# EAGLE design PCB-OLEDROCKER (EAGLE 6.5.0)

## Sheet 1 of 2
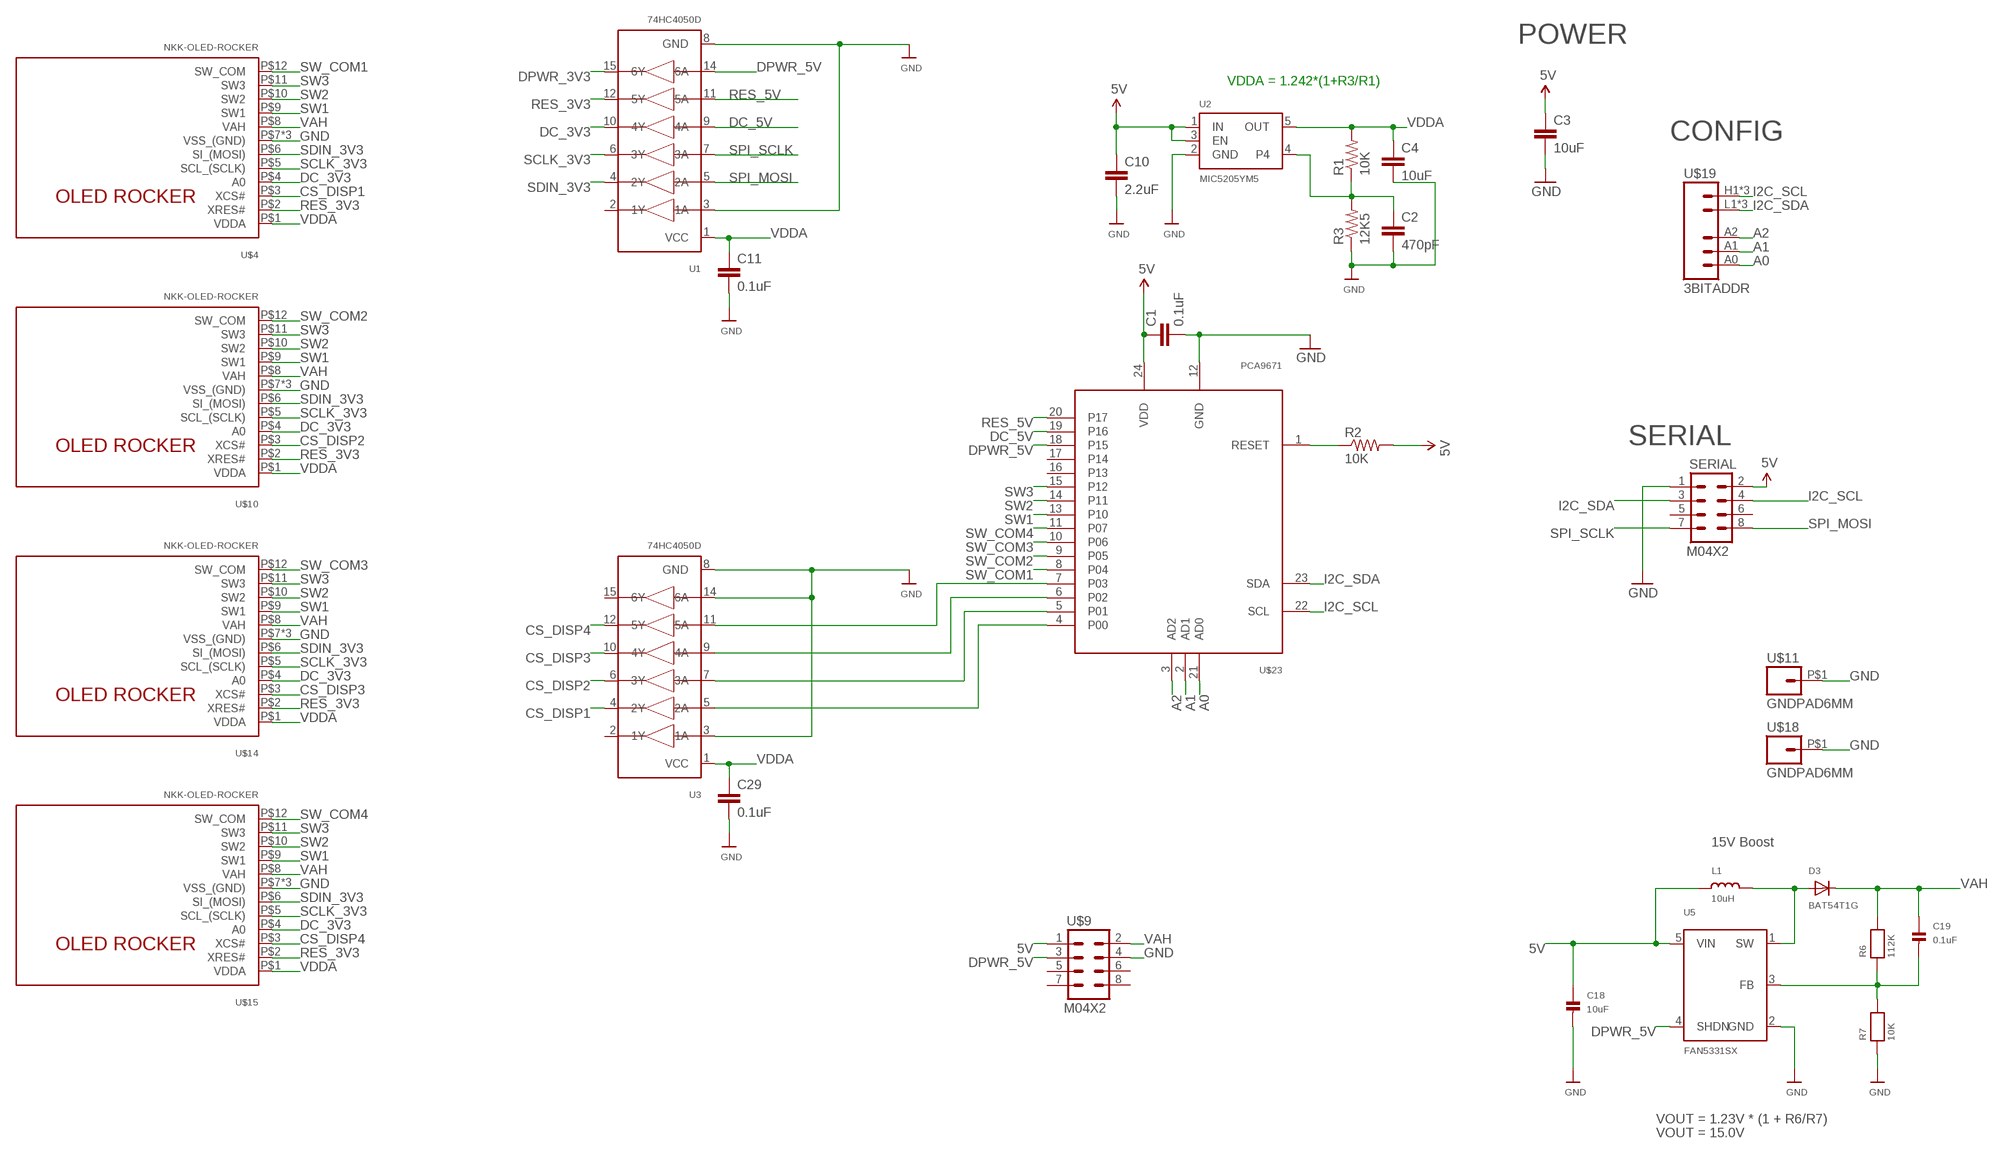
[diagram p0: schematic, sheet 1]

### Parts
C1  0.1uF  CAP0603-CAP  [0603-CAP]
C2  470pF  CAP0603-CAP  [0603-CAP]
C3  10uF  CAP0805  [0805]
C4  10uF  CAP0805  [0805]
C10  2.2uF  CAP0603-CAP  [0603-CAP]
C11  0.1uF  CAP0603-CAP  [0603-CAP]
C18  10uF  CAP_CERAMIC0805  [0805]
C19  0.1uF  CAP_CERAMIC0603  [0603]
C29  0.1uF  CAP0603-CAP  [0603-CAP]
D3  BAT54T1G  DIODESOD-123  [SOD-123]
L1  10uH  INDUCTOR  [INDUCTOR_1007]
R1  10K  RESISTOR0603-RES  [0603-RES]
R2  10K  RESISTOR0603-RES  [0603-RES]
R3  12K5  RESISTOR0603-RES  [0603-RES]
R6  112K  RESISTOR0603  [0603]
R7  10K  RESISTOR0603  [0603]
SERIAL  M04X2  [2X4]
U1  74HC4050D  74HC4050DTSSOP16  [TSSOP16]
U2  MIC5205YM5  VREG_SOT23-5  [SOT23-5]
U3  74HC4050D  74HC4050DTSSOP16  [TSSOP16]
U5  FAN5331SX  FAN5331  [SOT23-5]
U$4  NKK-OLED-ROCKER  [JST_BM12B-SURS]
U$9  M04X2  [2X4]
U$10  NKK-OLED-ROCKER  [JST_BM12B-SURS]
U$11  GNDPAD6MM  [3.2MMPAD6MM]
U$14  NKK-OLED-ROCKER  [JST_BM12B-SURS]
U$15  NKK-OLED-ROCKER  [JST_BM12B-SURS]
U$18  GNDPAD6MM  [3.2MMPAD6MM]
U$19  3BITADDR  [3BITADDR]
U$23  PCA9671  [TSSOP24]

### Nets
5V [Power]: C1.1 C3.1 C10.1 C18.1 L1.P$1 R2.2 SERIAL.2 U2.1(IN) U2.3(EN) U5.5(VIN) U$9.1 U$23.24(VDD)
A0: U$19.A0 U$23.21(AD0)
A1: U$19.A1 U$23.2(AD1)
A2: U$19.A2 U$23.3(AD2)
CS_DISP1: U3.4(2Y) U$4.P$3(XCS#)
CS_DISP2: U3.6(3Y) U$10.P$3(XCS#)
CS_DISP3: U3.10(4Y) U$14.P$3(XCS#)
CS_DISP4: U3.12(5Y) U$15.P$3(XCS#)
DC_3V3: U1.10(4Y) U$4.P$4(A0) U$10.P$4(A0) U$14.P$4(A0) U$15.P$4(A0)
DC_5V: U1.9(4A) U$23.19(P16)
DPWR_3V3: U1.15(6Y)
DPWR_5V [Power]: U1.14(6A) U5.4(SHDN) U$9.3 U$23.18(P15)
GND [Power]: C1.2 C2.2 C3.2 C4.2 C10.2 C11.2 C18.2 C29.2 R3.1 R7.1 SERIAL.1 U1.3(1A) U1.8(GND) U2.2(GND) U3.3(1A) U3.8(GND) U3.14(6A) U5.2(GND) U$4.P$7(VSS_(GND)) U$4.SUPPORT1(VSS_(GND)) U$4.SUPPORT2(VSS_(GND)) U$9.4 U$10.P$7(VSS_(GND)) U$10.SUPPORT1(VSS_(GND)) U$10.SUPPORT2(VSS_(GND)) U$11.P$1 U$14.P$7(VSS_(GND)) U$14.SUPPORT1(VSS_(GND)) U$14.SUPPORT2(VSS_(GND)) U$15.P$7(VSS_(GND)) U$15.SUPPORT1(VSS_(GND)) U$15.SUPPORT2(VSS_(GND)) U$18.P$1 U$23.12(GND)
I2C_SCL: SERIAL.4 U$19.H1(VCC) U$19.H2(VCC) U$19.H3(VCC) U$23.22(SCL)
I2C_SDA: SERIAL.3 U$19.L1(GND) U$19.L2(GND) U$19.L3(GND) U$23.23(SDA)
N$1: R2.1 U$23.1(RESET)
N$3: C2.1 R1.1 R3.2 U2.4
N$14 [Power]: D3.A L1.P$2 U5.1(SW)
N$15: C19.2 R6.1 R7.2 U5.3(FB)
N$29: U3.5(2A) U$23.4(P00)
N$30: U3.7(3A) U$23.5(P01)
N$31: U3.9(4A) U$23.6(P02)
N$32: U3.11(5A) U$23.7(P03)
RES_3V3: U1.12(5Y) U$4.P$2(XRES#) U$10.P$2(XRES#) U$14.P$2(XRES#) U$15.P$2(XRES#)
RES_5V: U1.11(5A) U$23.20(P17)
SCLK_3V3: U1.6(3Y) U$4.P$5(SCL_(SCLK)) U$10.P$5(SCL_(SCLK)) U$14.P$5(SCL_(SCLK)) U$15.P$5(SCL_(SCLK))
SDIN_3V3: U1.4(2Y) U$4.P$6(SI_(MOSI)) U$10.P$6(SI_(MOSI)) U$14.P$6(SI_(MOSI)) U$15.P$6(SI_(MOSI))
SPI_MOSI: SERIAL.8 U1.5(2A)
SPI_SCLK: SERIAL.7 U1.7(3A)
SW1: U$4.P$9(SW1) U$10.P$9(SW1) U$14.P$9(SW1) U$15.P$9(SW1) U$23.13(P10)
SW2: U$4.P$10(SW2) U$10.P$10(SW2) U$14.P$10(SW2) U$15.P$10(SW2) U$23.14(P11)
SW3: U$4.P$11(SW3) U$10.P$11(SW3) U$14.P$11(SW3) U$15.P$11(SW3) U$23.15(P12)
SW_COM1 [Power]: U$4.P$12(SW_COM) U$23.8(P04)
SW_COM2: U$10.P$12(SW_COM) U$23.9(P05)
SW_COM3: U$14.P$12(SW_COM) U$23.10(P06)
SW_COM4: U$15.P$12(SW_COM) U$23.11(P07)
VAH [Power]: C19.1 D3.C R6.2 U$4.P$8(VAH) U$9.2 U$10.P$8(VAH) U$14.P$8(VAH) U$15.P$8(VAH)
VDDA: C4.1 C11.1 C29.1 R1.2 U1.1(VCC) U2.5(OUT) U3.1(VCC) U$4.P$1(VDDA) U$10.P$1(VDDA) U$14.P$1(VDDA) U$15.P$1(VDDA)
Unconnected: SERIAL.5 SERIAL.6 U1.2(1Y) U3.2(1Y) U3.15(6Y) U$9.5 U$9.6 U$9.7 U$9.8 U$23.16(P13) U$23.17(P14)

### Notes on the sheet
- POWER
- VDDA = 1.242*(1+R3/R1)
- CONFIG
- SERIAL
- 15V Boost
- VOUT = 1.23V * (1 + R6/R7)
- VOUT = 15.0V

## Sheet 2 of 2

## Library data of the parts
C1-C4 C10 C11 C29 = SparkFun:CAP: Capacitor
C18 C19 = microbuilder:CAP_CERAMIC: Ceramic Capacitors
D3 = microbuilder:DIODE: Diode
L1 = microbuilder:INDUCTOR: Inductors
R1-R3 = SparkFun:RESISTOR: Resistor
R6 R7 = microbuilder:RESISTOR: Resistors
SERIAL U$9 = SparkFun:M04X2
U1 U3 = SKAARHOJ:74HC4050D: 6-channel level shifter 74HC4050D - 2V-6V Supply Digikey: 74HC4050D,653-ND Mouser: 771-74HC4050D-T
U2 = microbuilder:VREG_SOT23-5: SOT23-5 Fixed Voltage Regulators To better organise some of the SOT23-5 fixed voltage regulators in this library, this new part was created. Part Current Out V Out V In V Dropout Digikey Part No. ADP121 150mA 3.3V 3.4-5.5V 0.09V @ 150mA ADP121-AUJZ33R7CT-ND ADP121 150mA 3.0V 3.1-5.5V 0.09V @ 150mA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
U5 = microbuilder:FAN5331: FAN5331 - LED/OLED 20V Boost Converter Digikey: FAN5331SXCT-ND
U$4 U$10 U$14 U$15 = SKAARHOJ:NKK-OLED-ROCKER
U$11 U$18 = SKAARHOJ:GNDPAD
U$19 = SKAARHOJ:3BITADDR
U$23 = SKAARHOJ:PCA9671

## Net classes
0 default: width 0.203 mm, drill 0.305 mm, clearance 0.203 mm
1 Power: width 0.305 mm, drill 0.406 mm, clearance 0.203 mm

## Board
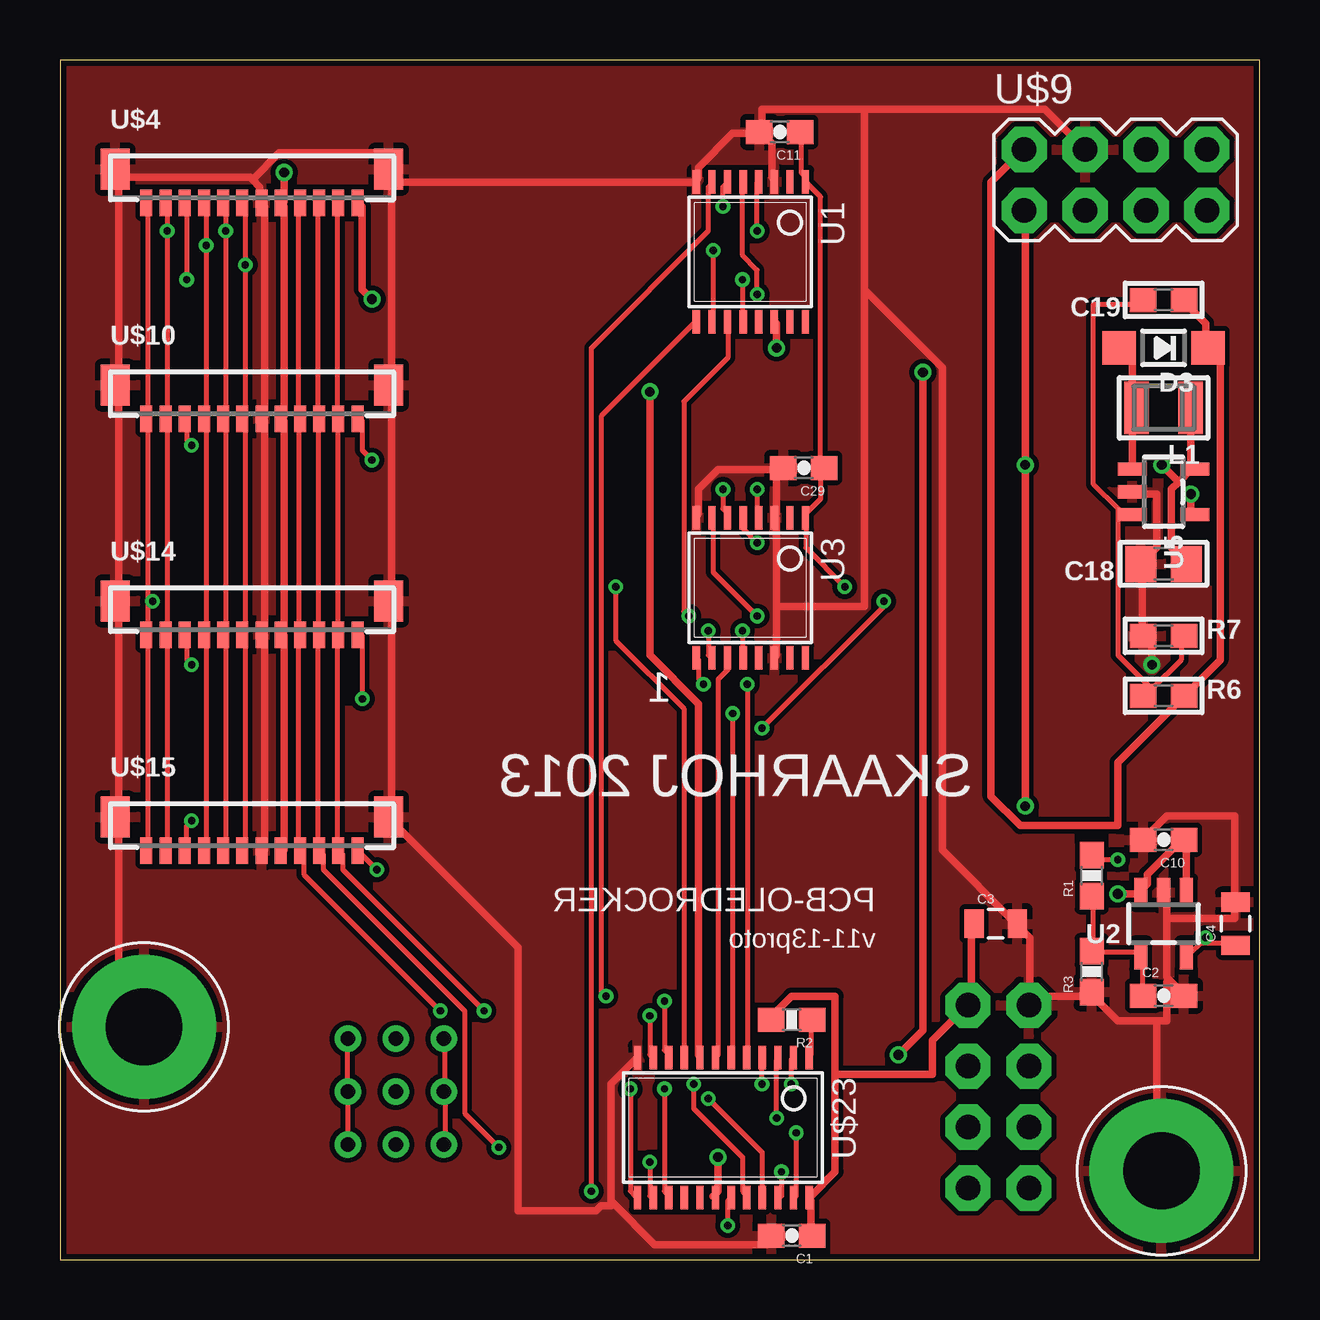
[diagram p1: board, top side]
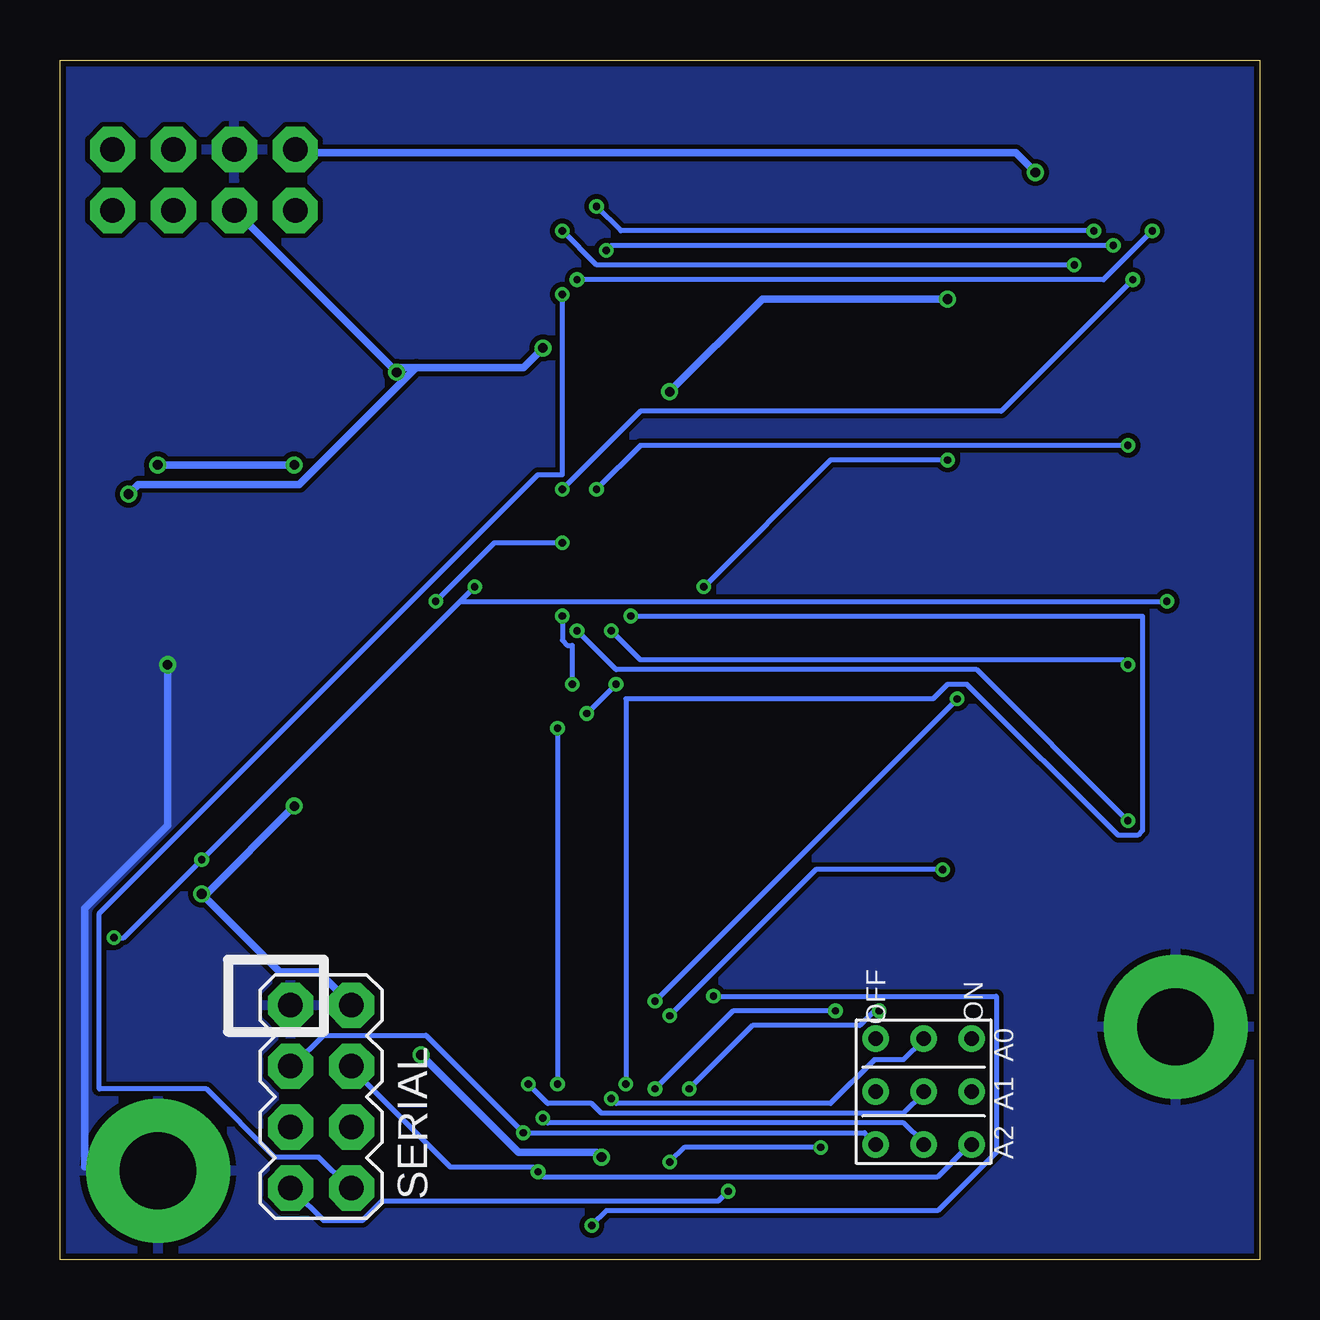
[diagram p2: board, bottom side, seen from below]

Size 50 x 50 mm. Coordinates in mm from the lower left corner, seen from the top.
Outline: 50,0 50,50 0,50 0,0 50,0
Copper layers (1*16): Top 0.035mm / dielectric 1.5mm / Bottom 0.035mm
Design rules "Fusion_eagle_rule_v1.1": minimum track width 6mil, minimum drill 12mil, track to track 6mil, track to pad 6mil, pad to pad 6mil, via to via 6mil, smd to smd 0mil, copper to edge 10mil, drill to drill 10mil, minimum pad ring 10mil, minimum via ring 6mil, stop-mask expansion 2mil, vias tented up to drill 100mil, thermal gap 10mil

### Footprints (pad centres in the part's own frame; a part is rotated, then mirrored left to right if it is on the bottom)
0603-CAP = smd 1.1 x 1: 1 -0.85,0; 2 0.85,0
0805 = smd 0.8 x 1.2: 1 -0.9,0; 2 0.9,0
0805' = smd 1.3 x 1.5: 1 -0.95,0; 2 0.95,0
0603 = smd 1.1 x 1: 1 -0.85,0; 2 0.85,0
SOD-123 = smd 1.4 x 1.4: A 1.85,0; C -1.85,0
INDUCTOR_1007 = smd 1.016 x 2.2: P$1 -1.127,0; P$2 1.127,0
0603-RES = smd 1.1 x 1: 1 -0.85,0; 2 0.85,0
2X4 = drill 1.016 pad 1.88 octagon: 1 -3.81,-1.27; 2 -3.81,1.27; 3 -1.27,-1.27; 4 -1.27,1.27; 5 1.27,-1.27; 6 1.27,1.27; 7 3.81,-1.27; 8 3.81,1.27
TSSOP16 = smd 0.305 x 0.991: 1 -3.575,-2.918; 2 -2.925,-2.918; 3 -2.275,-2.918; 4 -1.625,-2.918; 5 -0.975,-2.918; 6 -0.325,-2.918; 7 0.325,-2.918; 8 0.975,-2.918; 9 0.975,2.918; 10 0.325,2.918; 11 -0.325,2.918; 12 -0.975,2.918; 13 -1.625,2.918; 14 -2.275,2.918; 15 -2.925,2.918; 16 -3.575,2.918
SOT23-5 = smd 0.55 x 1.2: 1 -0.95,-1.3; 2 0,-1.3; 3 0.95,-1.3; 4 0.95,1.3; 5 -0.95,1.3
JST_BM12B-SURS = smd 0.5 x 1.1: P$1 -4.4,-1.95; P$2 -3.6,-1.95; P$3 -2.8,-1.95; P$4 -2,-1.95; P$5 -1.2,-1.95; P$6 -0.4,-1.95; P$7 0.4,-1.95; P$8 1.2,-1.95; P$9 2,-1.95; P$10 2.8,-1.95; P$11 3.6,-1.95; P$12 4.4,-1.95 | smd 1.2 x 1.7: SUPPORT1 5.7,-0.55; SUPPORT2 -5.7,-0.55
3.2MMPAD6MM = drill 3.2 pad 6: P$1 0,0
3BITADDR = drill 0.6: A0 -2.2,0; A1 0,0; A2 2.2,0; H1 -2.2,2; H2 0,2; H3 2.2,2; L1 -2.2,-2; L2 0,-2; L3 2.2,-2
TSSOP24 = smd 0.305 x 0.991: 1 -4.225,-2.918; 2 -3.575,-2.918; 3 -2.925,-2.918; 4 -2.275,-2.918; 5 -1.625,-2.918; 6 -0.975,-2.918; 7 -0.325,-2.918; 8 0.325,-2.918; 9 0.975,-2.918; 10 1.625,-2.918; 11 2.275,-2.918; 12 2.925,-2.918; 13 2.925,2.918; 14 2.275,2.918; 15 1.625,2.918; 16 0.975,2.918; 17 0.325,2.918; 18 -0.325,2.918; 19 -0.975,2.918; 20 -1.625,2.918; 21 -2.275,2.918; 22 -2.925,2.918; 23 -3.575,2.918; 24 -4.225,2.918

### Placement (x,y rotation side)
C1  30.5,1 180 top
C2  46,11 0 top
C3  39,14 0 top
C4  49,14 90 top
C10  46,17.5 180 top
C11  30,47 180 top
C18  10uF  [0805']  46,29 180 top
C19  46,40 180 top
C29  31,33 180 top
D3  46,38 180 top
L1  46,35.5 180 top
R1  43,16 90 top
R2  30.5,10 180 top
R3  43,12 90 top
R6  46,23.5 0 top
R7  46,26 0 top
SERIAL  39.12,6.79 270 bottom
U1  27.5,42 180 top
U2  46,14 180 top
U3  27.5,28 180 top
U5  46,32 270 top
U$4  8,46 0 top
U$9  44,45 0 top
U$10  8,37 0 top
U$11  45.92,3.7 0 top
U$14  8,28 0 top
U$15  8,19 0 top
U$18  3.5,9.7 0 top
U$19  14,7 270 bottom
U$23  27,5.5 180 top

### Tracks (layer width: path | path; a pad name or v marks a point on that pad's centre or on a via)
5V  (via drill 0.41)
  Top 0.305: C1.1 31.29,1.02 31.29,2.44 U$23.24 31.29,2.64 32.31,3.66 32.31,7.72 | 32.31,7.72 32.31,10.97 30.48,10.97 29.67,10.16 R2.2 | L1.P$1 47.14,35.36 47.14,33.12 U5.5 47.14,32.92 46.63,32.41 | 46.63,32.41 46.33,32.11 46.33,29.67 46.94,29.06 C18.1 | U2.1 46.94,15.44 46.94,17.48 C10.1 46.74,17.48 45.31,16.05 45.31,15.65 45.11,15.44 U2.3 44.91,15.24 v44.09,15.24 | C3.1 38,13.82 38,10.77 SERIAL.2 37.8,10.57 36.37,9.14 36.37,7.72 32.31,7.72 | v40.23,18.9 v40.23,33.12 40.23,43.69 U$9.1 | v45.92,33.12 46.63,32.41
  Bottom 0.305: SERIAL.2 38,10.77 39.22,11.99 40.84,11.99 v44.09,15.24 43.89,15.24 v40.23,18.9 | v40.23,33.12 v45.92,33.12
A0  (via drill 0.3)
  Top 0.203: v27.03,6.71 29.26,4.47 29.26,2.64 U$23.21
  Bottom 0.203: v27.03,6.71 26.82,6.5 17.88,6.5 16.05,8.33 14.83,8.33 14.02,9.14 U$19.A0
A1  (via drill 0.3)
  Top 0.203: v30.48,7.32 30.48,8.33 U$23.2
  Bottom 0.203: v30.48,7.32 29.67,6.5 27.84,6.5 27.43,6.1 14.83,6.1 14.02,6.91 U$19.A1
A2  (via drill 0.3)
  Top 0.203: v29.87,5.89 29.87,8.33 U$23.3
  Bottom 0.203: v29.87,5.89 29.67,5.69 14.83,5.69 14.02,4.88 U$19.A2
CS_DISP1  (via drill 0.3)
  Top 0.203: v29.06,32.11 29.06,31.09 U3.4 | v5.28,40.84 5.28,43.89 U$4.P$3
  Bottom 0.203: v29.06,32.11 25.81,35.36 10.77,35.36 v5.28,40.84
CS_DISP2  (via drill 0.3)
  Top 0.203: v27.64,32.11 27.64,31.29 27.84,31.09 U3.6 | v5.49,33.93 5.28,34.14 5.28,34.95 U$10.P$3
  Bottom 0.203: v27.64,32.11 25.81,33.93 v5.49,33.93
CS_DISP3  (via drill 0.3)
  Top 0.203: v27.03,26.21 27.03,25.2 U3.10 | v5.49,24.79 5.28,24.99 5.28,26.01 U$14.P$3
  Bottom 0.203: v27.03,26.21 25.81,24.99 5.69,24.99 v5.49,24.79
CS_DISP4  (via drill 0.3)
  Top 0.203: v28.45,26.21 28.45,25.2 U3.12 | v5.49,18.29 5.28,18.09 5.28,17.07 U$15.P$3
  Bottom 0.203: v28.45,26.21 26.82,24.59 11.79,24.59 v5.49,18.29
DC_3V3  (via drill 0.3)
  Top 0.203: U$15.P$4 6.1,17.07 6.1,26.01 U$14.P$4 6.1,26.21 6.1,34.95 U$10.P$4 6.1,35.15 v6.1,42.27 6.1,43.89 U$4.P$4 | v27.23,42.06 27.23,39.22 U1.10
  Bottom 0.203: v27.23,42.06 27.03,42.27 v6.1,42.27
DC_5V  (via drill 0.3)
  Top 0.203: v27.84,1.42 27.84,2.44 U$23.19 | v22.76,10.97 22.55,11.18 22.55,35.15 26.42,39.01 U1.9
  Bottom 0.203: v27.84,1.42 27.23,2.03 13.41,2.03 10.97,4.47 10.97,10.97 v22.76,10.97
DPWR_5V  (via drill 0.41)
  Top 0.305: v27.43,4.27 27.43,2.85 27.23,2.64 U$23.18 | v34.95,8.53 35.97,9.55 v35.97,36.98 | v29.87,38 29.87,39.01 U1.14 | v47.14,31.9 47.14,31.09 U5.4
  Bottom 0.305: v27.43,4.27 27.64,4.47 30.89,4.47 v34.95,8.53 | U$9.3 42.67,43.69 v35.97,36.98 35.97,37.19 35.15,37.19 | v29.87,38 30.68,37.19 35.15,37.19 | v47.14,31.9 46.74,32.31 40.03,32.31 35.15,37.19
GND  (via drill 0.41)
  Top 0.305: U$15.P$7 8.53,17.07 8.53,26.01 U$14.P$7 8.53,26.21 8.53,34.95 U$10.P$7 8.53,35.15 8.53,43.89 U$4.P$7 8.33,44.09 8.33,44.7 8.03,45.01 | 2.44,45.11 2.44,45.31 U$4.SUPPORT2 2.44,45.11 | 2.44,45.11 2.44,36.58 U$10.SUPPORT2 2.44,36.37 2.44,27.64 U$14.SUPPORT2 2.44,27.43 2.44,18.49 U$15.SUPPORT2 2.44,18.29 2.44,10.77 3.45,9.75 U$18.P$1 | 8.03,45.01 7.92,45.11 2.44,45.11 | 40.44,10.97 42.88,10.97 R3.1 43.08,10.97 44.09,9.96 45.72,9.96 | 40.44,10.97 40.44,10.77 SERIAL.1 40.44,10.97 | 40.44,10.97 40.44,13.41 40.03,13.82 C3.2 39.83,14.02 36.78,17.07 36.78,37.19 33.53,40.44 | 46.23,11.68 46.13,11.79 46.13,14.22 | 46.23,11.68 46.74,11.18 C2.2 | 46.13,14.22 46.13,15.24 U2.2 | C10.2 45.31,17.68 46.13,18.49 48.97,18.49 48.97,15.04 C4.2 48.97,14.83 48.97,14.22 46.13,14.22 | 45.72,9.96 46.13,9.96 46.13,11.58 46.23,11.68 | U5.2 44.7,31.9 45.72,31.9 45.72,29.67 45.11,29.06 C18.2 45.11,28.85 45.11,26.01 R7.1 45.31,25.81 45.52,25.6 v45.52,24.79 | 45.72,9.96 45.72,3.86 U$11.P$1 | 23.06,2.34 24.79,0.61 29.46,0.61 29.46,0.81 C1.2 | 23.06,2.34 22.96,2.44 22.96,7.32 23.98,8.33 U$23.12 | 29.87,27.23 29.87,30.89 U3.3 29.87,31.09 29.87,32.92 | 29.87,27.23 29.87,25.2 U3.14 | 29.87,32.92 30.07,32.92 C29.2 29.87,32.92 | 29.87,32.92 27.43,32.92 26.62,32.11 26.62,31.09 U3.8 | C11.2 29.06,46.94 28.04,46.94 26.62,45.52 26.62,45.11 U1.8 26.42,44.91 13.82,44.91 | U1.3 29.67,45.11 29.67,46.53 29.26,46.94 C11.2 | 13.82,44.91 13.82,45.31 U$4.SUPPORT1 | 13.82,44.91 13.82,36.58 U$10.SUPPORT1 13.82,36.37 13.82,27.64 U$14.SUPPORT1 13.82,27.43 13.82,18.49 U$15.SUPPORT1 13.82,18.29 19.1,13.01 19.1,2.03 22.35,2.03 22.55,2.23 22.96,2.23 23.06,2.34
  Top 0.305: 13.82,44.91 U$4.SUPPORT1 | 33.53,47.95 29.26,47.95 29.26,47.14 C11.2 | 33.53,47.95 41.05,47.95 42.67,46.33 U$9.4 | 29.87,27.23 33.53,27.23 33.53,40.44 | 33.53,47.95 33.53,40.44 | 8.03,45.01 9.14,46.13 13.61,46.13 13.61,45.52 U$4.SUPPORT1
  Bottom 0.305: v45.52,24.79 45.52,18.09 48.97,14.63 48.97,3.86 45.92,3.86 U$11.P$1
  pour Top: 0,0 50,0 50,50 0,50
  pour Bottom: 0,0 50,0 50,50 0,50
I2C_SCL  (via drill 0.3)
  Top 0.203: U$19.H3 11.99,4.88 11.99,6.91 U$19.H2 11.99,7.11 11.99,9.14 U$19.H1 | v30.07,3.66 30.07,2.64 U$23.22
  Bottom 0.203: SERIAL.4 37.8,7.92 33.73,3.86 30.28,3.86 v30.07,3.66 29.87,3.45 13.41,3.45 12.19,4.67 U$19.H3
I2C_SDA  (via drill 0.3)
  Top 0.203: U$19.L3 16.05,4.88 16.05,6.91 U$19.L2 16.05,7.11 16.05,9.14 U$19.L1 | v30.68,5.28 30.68,2.64 U$23.23
  Bottom 0.203: SERIAL.3 40.23,8.13 39.01,9.35 34.75,9.35 v30.68,5.28 16.46,5.28 16.05,4.88 U$19.L3
N$1
  Top 0.203: U$23.1 31.29,8.53 31.29,9.96 R2.1
N$3
  Top 0.203: C2.1 45.11,11.18 45.11,12.6 U2.4 44.91,12.8 43.08,12.8 R3.2 43.08,13.01 43.08,15.04 R1.1
N$14
  Top 0.305: U5.1 44.7,33.12 44.7,35.36 L1.P$2 44.7,35.56 44.7,37.59 44.3,38 D3.A
N$15
  Top 0.203: 45.52,23.77 46.74,24.99 46.74,25.81 R7.2 | 45.52,23.77 45.31,23.57 R6.1 45.52,23.77 | 44.09,31.29 44.5,30.89 U5.3 | 44.09,31.29 43.08,32.31 43.08,39.83 45.11,39.83 C19.2 | 45.52,23.77 44.09,25.2 44.09,31.29
N$29  (via drill 0.3)
  Top 0.203: v29.26,7.32 29.26,8.33 U$23.4 | v29.26,22.15 34.34,27.23 v34.34,27.43 | v29.06,29.87 28.45,30.48 28.45,30.89 U3.5
  Bottom 0.203: v29.26,22.15 v29.26,7.32 | v34.34,27.43 31.9,29.87 v29.06,29.87
N$30  (via drill 0.3)
  Top 0.203: v28.65,23.98 28.65,8.53 U$23.5 | v29.06,26.82 27.23,28.65 27.23,30.89 U3.7
  Bottom 0.203: v28.65,23.98 28.65,25.6 28.85,25.6 29.06,25.81 v29.06,26.82
N$31  (via drill 0.3)
  Top 0.203: v28.04,22.76 28.04,8.53 U$23.6 | v26.82,23.98 26.62,24.18 26.62,24.99 U3.9
  Bottom 0.203: v26.82,23.98 v28.04,22.76
N$32
  Top 0.203: U$23.7 27.43,8.53 27.43,24.18 27.84,24.59 27.84,24.99 U3.11
RES_3V3  (via drill 0.3)
  Top 0.203: U$15.P$2 4.47,17.07 4.47,26.01 U$14.P$2 4.47,26.21 4.47,34.95 U$10.P$2 4.47,35.15 v4.47,42.88 4.47,43.89 U$4.P$2 | v28.45,40.84 28.45,39.22 U1.12
  Bottom 0.203: v28.45,40.84 6.5,40.84 v4.47,42.88
RES_5V  (via drill 0.3)
  Top 0.203: v26.42,7.32 26.42,6.3 28.45,4.27 28.45,2.85 28.65,2.64 U$23.20 | v26.21,26.82 26.01,27.03 26.01,35.76 27.84,37.59 27.84,39.01 U1.11
  Bottom 0.203: v26.42,7.32 26.42,23.37 13.61,23.37 13.01,23.98 12.19,23.98 5.89,17.68 5.08,17.68 4.88,17.88 4.88,26.82 v26.21,26.82
SCLK_3V3  (via drill 0.3)
  Top 0.203: U$15.P$5 6.91,17.07 6.91,26.01 U$14.P$5 6.91,26.21 6.91,34.95 U$10.P$5 6.91,35.15 v6.91,42.88 6.91,43.89 U$4.P$5 | v27.64,43.89 27.64,44.7 27.84,44.91 U1.6
  Bottom 0.203: v27.64,43.89 26.62,42.88 v6.91,42.88
SDIN_3V3  (via drill 0.3)
  Top 0.203: U$15.P$6 7.72,17.07 7.72,26.01 U$14.P$6 7.72,26.21 7.72,34.95 U$10.P$6 7.72,35.15 v7.72,41.45 7.72,43.89 U$4.P$6 | v29.06,42.88 29.06,44.91 U1.4
  Bottom 0.203: v29.06,42.88 27.64,41.45 v7.72,41.45
SPI_MOSI  (via drill 0.3)
  Top 0.203: v29.06,40.23 29.06,41.25 28.45,41.86 28.45,44.91 U1.5
  Bottom 0.203: v29.06,40.23 29.06,32.72 30.07,32.72 48.36,14.43 48.36,7.11 43.89,7.11 41.05,4.27 39.22,4.27 38,3.05 SERIAL.8
SPI_SCLK  (via drill 0.3)
  Top 0.203: v22.15,2.85 22.15,38 27.03,42.88 27.03,44.7 27.23,44.91 U1.7
  Bottom 0.203: v22.15,2.85 22.55,2.44 36.58,2.44 37.39,1.63 39.01,1.63 40.23,2.85 SERIAL.7
SW1  (via drill 0.3)
  Top 0.203: U$4.P$9 9.96,43.89 9.96,35.15 U$10.P$9 9.96,34.95 9.96,26.21 U$14.P$9 9.96,26.01 9.96,17.07 U$15.P$9 10.16,16.87 10.16,16.05 v15.85,10.36 | v23.77,7.11 23.77,2.85 23.98,2.64 U$23.13
  Bottom 0.203: v23.77,7.11 21.13,9.75 16.66,9.75 16.05,10.36 v15.85,10.36
SW2  (via drill 0.3)
  Top 0.203: U$4.P$10 10.77,43.89 10.77,35.15 U$10.P$10 10.77,34.95 10.77,26.21 U$14.P$10 10.77,26.01 10.77,17.07 U$15.P$10 10.97,16.87 10.97,16.26 16.87,10.36 16.87,6.1 v18.29,4.67 | v24.59,4.06 24.59,2.64 U$23.14
  Bottom 0.203: v24.59,4.06 23.98,4.67 v18.29,4.67
SW3  (via drill 0.3)
  Top 0.203: U$4.P$11 11.58,43.89 11.58,35.15 U$10.P$11 11.58,34.95 11.58,26.21 U$14.P$11 11.58,26.01 11.58,17.07 U$15.P$11 11.79,16.87 11.79,16.26 v17.68,10.36 | v25.2,7.11 25.2,2.85 25.4,2.64 U$23.15
  Bottom 0.203: v25.2,7.11 21.95,10.36 v17.68,10.36
SW_COM1  (via drill 0.41)
  Top 0.305: v24.59,36.17 24.59,25.2 26.62,23.16 26.62,8.53 U$23.8 | v13.01,40.03 12.6,40.44 12.6,43.89 U$4.P$12
  Bottom 0.305: v24.59,36.17 20.73,40.03 v13.01,40.03
SW_COM2  (via drill 0.3)
  Top 0.203: v23.16,28.04 23.16,25.81 26.01,22.96 26.01,8.53 U$23.9 | v13.01,33.33 12.6,33.73 12.6,34.95 U$10.P$12
  Bottom 0.203: v23.16,28.04 17.88,33.33 v13.01,33.33
SW_COM3  (via drill 0.3)
  Top 0.203: v25.2,10.77 25.2,8.74 25.4,8.53 U$23.10 | v12.6,23.37 12.6,26.01 U$14.P$12
  Bottom 0.203: v12.6,23.37 v25.2,10.77
SW_COM4  (via drill 0.3)
  Top 0.203: v24.59,10.16 24.59,8.53 U$23.11 | v13.21,16.26 12.6,16.87 U$15.P$12
  Bottom 0.203: v24.59,10.16 18.49,16.26 v13.21,16.26
VAH  (via drill 0.41)
  Top 0.305: U$15.P$8 9.35,17.07 9.35,26.01 U$14.P$8 9.35,26.21 9.35,34.95 U$10.P$8 9.35,35.15 9.35,43.89 U$4.P$8 9.35,44.09 v9.35,45.31 | C19.1 46.94,39.83 47.75,39.01 47.75,38.2 D3.C 47.95,38 48.36,37.59 48.36,24.99 46.94,23.57 R6.2 46.74,23.37 44.09,20.73 44.09,18.09 40.03,18.09 38.81,19.3 38.81,44.91 40.03,46.13 U$9.2
  Bottom 0.305: v9.35,45.31 10.16,46.13 40.03,46.13 U$9.2
VDDA  (via drill 0.3)
  Top 0.203: U$15.P$1 3.66,17.07 3.66,26.01 U$14.P$1 3.66,26.21 3.66,27.43 | U$4.P$1 3.66,43.89 3.66,35.15 U$10.P$1 3.66,34.95 3.66,27.43 | v44.09,16.66 43.08,16.66 R1.2 | 47.55,13.21 47.14,12.8 U2.5 | 47.55,13.21 48.97,13.21 C4.1 | 47.55,13.21 v47.75,13.41 | C11.1 30.89,46.94 30.89,45.31 31.09,45.11 U1.1 31.09,44.91 31.7,44.3 31.7,33.12 C29.1 31.7,32.92 31.7,31.7 31.09,31.09 U3.1 31.09,30.89 31.09,29.67 v32.72,28.04 | v3.86,27.43 3.66,27.43
  Bottom 0.203: v47.75,13.41 47.35,13.41 v44.09,16.66 33.33,27.43 | v32.72,28.04 33.33,27.43 | 33.33,27.43 v3.86,27.43

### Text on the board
_tsilk: 1 | SKAARHOJ 2013 | PCB-OLEDROCKER | v11-13proto

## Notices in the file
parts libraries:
SparkFun: Licensing: CC v3.0 Share-Alike You are welcome to use this library for commercial purposes.
